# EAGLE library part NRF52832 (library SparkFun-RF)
Nordic nRF52832 Bluetooth Smart/ANT/2.4GHz RF SoC The nRF52832 SoC is a powerful, highly flexible ultra-low power multiprotocol SoC ideally suited for Bluetooth® Smart ANT and 2.4GHz ultra low-power wireless applications. The nRF52832 SoC is built around a 32-bit ARM® Cortex™-M4F CPU with 512kB + 64kB RAM. The embedded 2.4GHz transceiver supports Bluetooth Smart, ANT and proprietary 2.4 GHz protocol stack. It is on air compatible with the nRF51 Series, nRF24L and nRF24AP Series products from Nordic Semiconductor. Datasheet SparkFun Products: SparkFun nRF52832 Breakout
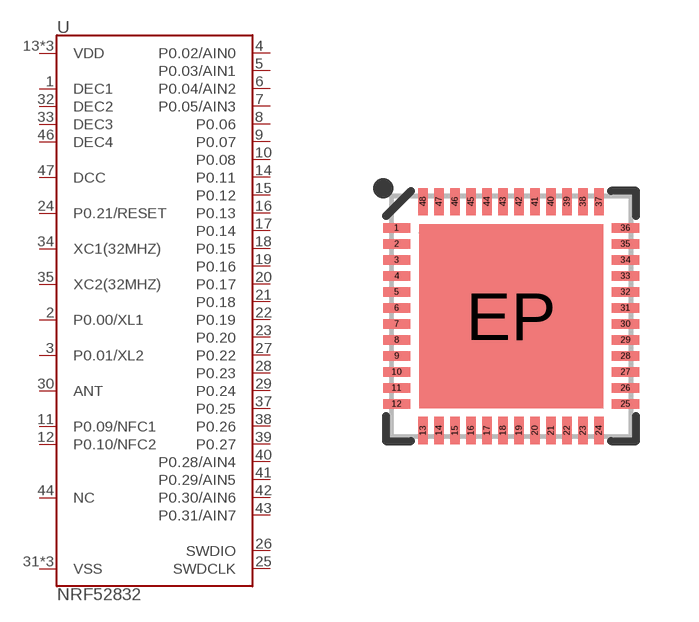
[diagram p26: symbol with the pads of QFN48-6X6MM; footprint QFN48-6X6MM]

Designator prefix U

## NRF52832 (PROD_ID: IC-13460)  [QFN48-6X6MM]
1  DEC1
2  P0.00/XL1
3  P0.01/XL2
4  P0.02/AIN0
5  P0.03/AIN1
6  P0.04/AIN2
7  P0.05/AIN3
8  P0.06
9  P0.07
10  P0.08
11  P0.09/NFC1
12  P0.10/NFC2
13  VDD
14  P0.11
15  P0.12
16  P0.13
17  P0.14
18  P0.15
19  P0.16
20  P0.17
21  P0.18
22  P0.19
23  P0.20
24  P0.21/RESET
25  SWDCLK
26  SWDIO
27  P0.22
28  P0.23
29  P0.24
30  ANT
31  VSS
32  DEC2
33  DEC3
34  XC1(32MHZ)
35  XC2(32MHZ)
36  VDD
37  P0.25
38  P0.26
39  P0.27
40  P0.28/AIN4
41  P0.29/AIN5
42  P0.30/AIN6
43  P0.31/AIN7
44  NC
45  VSS
46  DEC4
47  DCC
48  VDD
EP  VSS

## Footprint QFN48-6X6MM (pad centres in mm)
QFN-48 pin 6x6mm Specifications: Pin count: 48 Area: 6x6mm Datasheet referenced for footprint Example device(s): nRF52832
smd 0.68 x 0.23: 1 -2.86,2.2; 2 -2.86,1.8; 3 -2.86,1.4; 4 -2.86,1; 5 -2.86,0.6; 6 -2.86,0.2; 7 -2.86,-0.2; 8 -2.86,-0.6; 9 -2.86,-1; 10 -2.86,-1.4; 11 -2.86,-1.8; 12 -2.86,-2.2; 25 2.86,-2.2; 26 2.86,-1.8; 27 2.86,-1.4; 28 2.86,-1; 29 2.86,-0.6; 30 2.86,-0.2; 31 2.86,0.2; 32 2.86,0.6; 33 2.86,1; 34 2.86,1.4; 35 2.86,1.8; 36 2.86,2.2
smd 0.23 x 0.68: 13 -2.2,-2.86; 14 -1.8,-2.86; 15 -1.4,-2.86; 16 -1,-2.86; 17 -0.6,-2.86; 18 -0.2,-2.86; 19 0.2,-2.86; 20 0.6,-2.86; 21 1,-2.86; 22 1.4,-2.86; 23 1.8,-2.86; 24 2.2,-2.86; 37 2.2,2.86; 38 1.8,2.86; 39 1.4,2.86; 40 1,2.86; 41 0.6,2.86; 42 0.2,2.86; 43 -0.2,2.86; 44 -0.6,2.86; 45 -1,2.86; 46 -1.4,2.86; 47 -1.8,2.86; 48 -2.2,2.86
smd 4.6 x 4.6: EP 0,0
